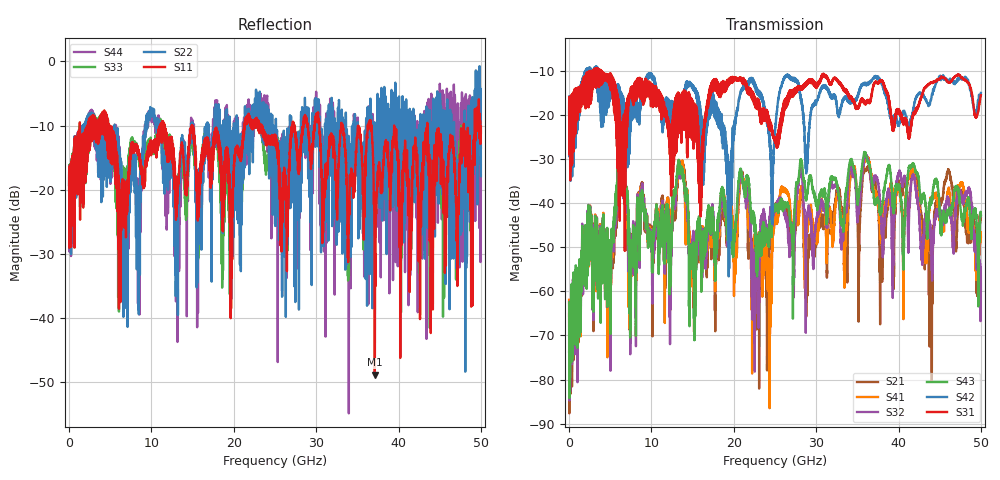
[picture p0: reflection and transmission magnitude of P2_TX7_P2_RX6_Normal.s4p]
!Keysight Technologies,N5225B,MY57041031,A.13.20.10
!Date: Friday, May 31, 2019 11:36:28
!Correction: S11(Full 4 Port(1,2,3,4))
!S12(Full 4 Port(1,2,3,4))
!S13(Full 4 Port(1,2,3,4))
!S14(Full 4 Port(1,2,3,4))
!S21(Full 4 Port(1,2,3,4))
!S22(Full 4 Port(1,2,3,4))
!S23(Full 4 Port(1,2,3,4))
!S24(Full 4 Port(1,2,3,4))
!S31(Full 4 Port(1,2,3,4))
!S32(Full 4 Port(1,2,3,4))
!S33(Full 4 Port(1,2,3,4))
!S34(Full 4 Port(1,2,3,4))
!S41(Full 4 Port(1,2,3,4))
!S42(Full 4 Port(1,2,3,4))
!S43(Full 4 Port(1,2,3,4))
!S44(Full 4 Port(1,2,3,4))
!S4P File: Measurements: <S11,S12,S13,S14>,
!<S21,S22,S23,S24>,
!<S31,S32,S33,S34>,
!<S41,S42,S43,S44>:
# Hz S  dB  R 50.0
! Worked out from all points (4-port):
!   5000 points, 10 MHz to 50 GHz, reference 50 ohm
!   strongest paths, dB at 10 MHz, 12.51 GHz, 25.01 GHz, 37.51 GHz, 50 GHz:
!     S31: -19.6, -22.5, -25.7, -12.7, -15.4
!     S42: -19.3, -16.9, -23.7, -11.4, -14.9
!     S43: -62.5, -44.8, -40.7, -39.1, -42.6
!     S32: -73.6, -46.0, -40.9, -35.1, -59.5
!     S41: -61.9, -46.1, -42.0, -40.3, -47.6
!     S21: -65.1, -46.4, -40.6, -40.4, -43.0
!   lowest |S11| = -48.8 dB at 37.12 GHz (marker M1), VSWR 1.01, Z = 49.9 - j0.331 ohm
!   |S11| at or under -10 dB: 4.911 GHz to 11.03 GHz (6.119 GHz wide, 76.8 % of centre); 14.96 GHz to 21.26 GHz (6.298 GHz wide, 34.8 % of centre); 43.5 GHz to 47.92 GHz (4.413 GHz wide, 9.65 % of centre)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
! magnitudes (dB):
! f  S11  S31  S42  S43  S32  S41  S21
! 10 MHz  -20.2  -19.6  -19.3  -62.5  -73.6  -61.9  -65.1
! 6.19 GHz  -37.4  -20.5  -16.2  -26.9  -27.3  -27.3  -27.8
! 7.47 GHz  -13.8  -15.1  -15.5  -61.1  -60.7  -57.6  -58.1
! 13.55 GHz  -14.1  -16.7  -18.1  -31.6  -32.5  -30.7  -31.4
! 22.9 GHz  -9.2  -18.5  -14.6  -50.5  -57.4  -47.9  -55.7
! 37.12 GHz  -48.8  -12.6  -11.4  -40.1  -34.1  -37.4  -34.8
! 50 GHz  -11.1  -15.4  -14.9  -42.6  -59.5  -47.6  -43.0
